{attribute 'no_assign'}
FUNCTION_BLOCK FB_IEDServerSession IMPLEMENTS I_ScsmAbortIndEventSink, I_ScsmAssociateIndEventSink, I_ScsmReleaseIndEventSink
VAR_INPUT
	fbConnection		: FB_iec61850ConnectionClass := (ipAbortInd:=THIS^, ipAssociateInd:=THIS^, ipReleaseInd:=THIS^);
END_VAR
VAR
	_bAbort				: BOOL; (* Rising edge activates AbortReq() command execution *)
	_bDisconnect		: BOOL; (* Rising edge activates ReleaseReq() command execution *)
	
	state				: BYTE;
	eState				: E_AsyncEnvironmentState; (* Environment state *)
	eLinkStatus			: E_ScsmLinkStatus; (* Network adapter link status *)
	bBusy				: BOOL; (* If TRUE => command execution is busy *)
	bSuccess			: BOOL;
	ipResult			: I_AsyncServiceResultClass;
	sLastErrorResult	: T_MaxString;
	fbAbortReason		: FB_ServiceErrorClass := (stError:=SUCCESS_EVENT);
	sLastAbortReason	: T_MaxString;
END_VAR

fbConnection.Execute();
eState:= fbConnection.eState;
eLinkStatus:= fbConnection.eLinkStatus;

(* Execute control model control block implementations *)
fbIED.IEDMUnn.LLN0.Mod_.fbControl.Execute(); (* ctlModel is "status-only", therefore object is not controllable *)

CASE state OF
	0: (* Initial state *)
		IF _bAbort THEN (* Abort connection => execute AbortReq() command *)
			_bAbort:= FALSE;
			bSuccess:= fbConnection.AbortReq(ipReason:=fbAbortReason, ipSink:=0, ipResult=>ipResult);
			state:= SEL(bSuccess, 100, 1);
		ELSIF eState = E_AsyncEnvironmentState.Established AND _bDisconnect THEN (* Close/release connection => execute ReleaseReq() command *)
			_bDisconnect:= FALSE;
			bSuccess:= fbConnection.ReleaseReq(ipSink:=0, ipResult=>ipResult);
			state:= SEL(bSuccess, 100, 1);
		ELSIF eState = E_AsyncEnvironmentState.Established THEN (* Connection established => exchange IED data *)
			state:= 10;
		END_IF
		_bDisconnect:= FALSE;
		(*==================================================================================================================================================================*)
	1: (* Wait for AbortReq() or ReleaseReq() command completion *)
		IF ipResult <> 0 THEN
			ipResult.Execute();
			IF NOT (bBusy:=ipResult.IsBusy()) THEN
				state:= SEL(ipResult.IsCompleted(), 100(* failed or aborted *), 0(* succeeded *));
			END_IF
		END_IF
		(*==================================================================================================================================================================*)
	10: (* connection established *)
		state:= 0;
		(*==================================================================================================================================================================*)
	100: (* Error state *)
		state:= 0;
		IF ipResult <> 0 THEN
			sLastErrorResult:= ipResult.Dump();
		END_IF
END_CASE

PROPERTY bAbort : BOOL
SET
_bAbort:= bAbort;
END_SET
END_PROPERTY

PROPERTY bDisconnect : BOOL
SET
_bDisconnect:= bDisconnect;
END_SET
END_PROPERTY

{attribute 'analysis' := '-33'}
(* This method receives IEC61850::Abort.ind primitive. *)
METHOD OnAbortInd
VAR_INPUT
	ipAA		: I_ScsmAssociationClass; (* Application association. If = 0 => optional. *)
	bPAbort		: BOOL; (* TRUE => P-Abort.request(), issued by provider, FALSE => Abort.request(), issued by user. *)
	ipReason	: I_ServiceErrorClass; (* Abort reason. *)
	ipData		: I_BaseStreamClass; (* Optional data. If = 0 => default, no data. *)
END_VAR
VAR
END_VAR
IF ipReason <> 0 THEN
	sLastAbortReason:= ipReason.Dump();
END_IF
END_METHOD

{attribute 'analysis' := '-33'}
(* This method receives IEC61850::Associate.ind primitive. *)
METHOD OnAssociateInd : BOOL
VAR_INPUT
	ipAA			: I_ScsmAssociationClass; (* Application association. If = 0 => optional. *)
END_VAR
VAR_OUTPUT
	ipResult		: I_AsyncServiceResultClass; (* Interface pointer to service state and result information *)
END_VAR
VAR
END_VAR
sLastAbortReason:= '';
sLastErrorResult:= '';
OnAssociateInd:= fbConnection.AssociateRsp(ipResult=>ipResult);
END_METHOD

{attribute 'analysis' := '-33'}
(* This method receives IEC61850::Release.ind primitive. *)
METHOD OnReleaseInd : BOOL
VAR_INPUT
	ipAA	: I_ScsmAssociationClass; (* Application association. If = 0 => optional. *)
END_VAR
VAR_OUTPUT
	ipResult: I_AsyncServiceResultClass; (* Interface pointer to service state and result information *)
END_VAR
VAR
END_VAR
OnReleaseInd:= fbConnection.ReleaseRsp(ipResult=>ipResult);
END_METHOD

END_FUNCTION_BLOCK
